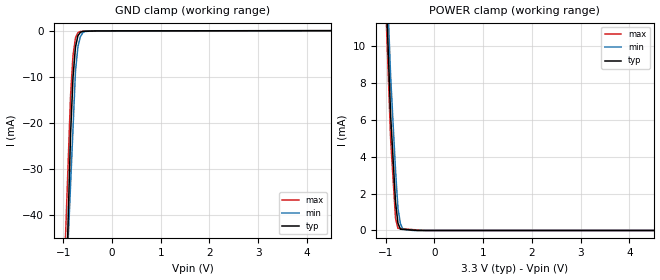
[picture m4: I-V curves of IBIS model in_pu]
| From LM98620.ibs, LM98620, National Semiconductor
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[Model] in_pu
Model_type Input
Vinl = 800.000mV
Vinh = 2.00000V
C_comp 642.000fF 588.000fF 642.000fF
| variable typ   min   max
[Voltage Range] 3.30000V 3.00000V 3.60000V
[POWER Clamp Reference] 3.30000V 3.00000V 3.60000V
[GND Clamp Reference] 0.00000V 0.00000V 0.00000V
[Temperature Range]   25   70   0
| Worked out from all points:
|   GND clamp passes 1 mA (typ) near -0.69 V on its own axis
|   POWER clamp passes 1 mA (typ) near -0.78 V on its own axis
[GND Clamp]
-3.3V     -934.3mA   -633.5mA   -739mA
-850mV    -22.45mA   -33.38mA   -14.05mA
-800mV    -10.09mA   -21.14mA   -5.353mA
-750mV    -3.595mA   -8.89mA    -1.573mA
-700mV    -1.092mA   -3.521mA   -430.8uA
-650mV    -364.6uA   -1.335mA   -148.8uA
-600mV    -122.1uA   -435.6uA   -131.9uA
-550mV    -107.7uA   -152uA     -115uA
-325mV    -42.61uA   -50.18uA   -38.89uA
-300mV    -35.38uA   -38.87uA   -38.63uA
-275mV    -35.14uA   -27.56uA   -38.37uA
6.6V      33.14uA    31.71uA    33.11uA
[POWER Clamp]
-3.3V     205mA      182.2mA    177.8mA
-1.05V    16.95mA    18.63mA    15.75mA
-900mV    6.237mA    8.344mA    4.953mA
-800mV    1.541mA    3.269mA    666.7uA
-750mV    395.8uA    1.206mA    112.9uA
-700mV    69.46uA    375.3uA    102.1uA
-650mV    59.54uA    78.22uA    91.39uA
-450mV    19.85uA    0A         48.38uA
-175mV    0A         0A         0A
6.6V      0A         0A         0A
